ORGANIZATION_BLOCK "Blocco Organizzativo"
TITLE = "Main Program Sweep (Cycle)"
AUTHOR : MassimoZ
FAMILY : NovaSrl
VERSION : 0.1


VAR_TEMP
  OB1_EV_CLASS : BYTE ;	//Bits 0-3 = 1 (Coming event), Bits 4-7 = 1 (Event class 1)
  OB1_SCAN_1 : BYTE ;	//1 (Cold restart scan 1 of OB 1), 3 (Scan 2-n of OB 1)
  OB1_PRIORITY : BYTE ;	//1 (Priority of 1 is lowest)
  OB1_OB_NUMBR : BYTE ;	//1 (Organization block 1, OB1)
  OB1_RESERVED_1 : BYTE ;	//Reserved for system
  OB1_RESERVED_2 : BYTE ;	//Reserved for system
  OB1_PREV_CYCLE : INT ;	//Cycle time of previous OB1 scan (milliseconds)
  OB1_MIN_CYCLE : INT ;	//Minimum cycle time of OB1 (milliseconds)
  OB1_MAX_CYCLE : INT ;	//Maximum cycle time of OB1 (milliseconds)
  OB1_DATE_TIME : DATE_AND_TIME ;	//Date and time OB1 started
END_VAR
BEGIN
NETWORK
TITLE =Condizioni di Sicurezza OK
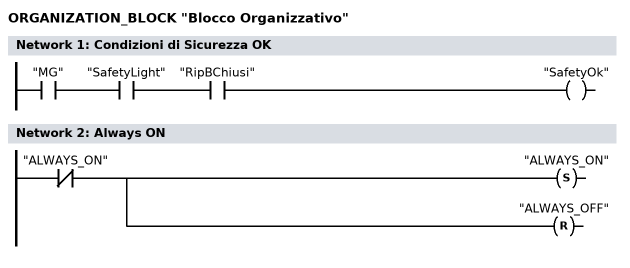
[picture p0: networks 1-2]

      U     "MG";
      U     "SafetyLight";
      U     "RipBChiusi";
      =     "SafetyOk";
NETWORK
TITLE =Always ON

      UN    "ALWAYS_ON";
      S     "ALWAYS_ON";
      R     "ALWAYS_OFF";
NETWORK
TITLE =Gestione Consensi

      UC    "Gest Consensi 2ndCC";

NETWORK
TITLE =Gestione Ciclo Automatico
//FC 49 gestisce il quadro di Ferrazza , mentre il FC50 gestisce, se abilitato,
//il quadro controllo corti tradizionale con slaughter STS
      UC    "Gest Auto 2ndCC";
// UC    "Gest Auto STS"
NETWORK
TITLE =Gestione Avvisi e Allarmi

      UC    "Gest Avvisi Allarmi";

NETWORK
TITLE =Gestione Interfaccia

      UC    "Gest Interfaccia";

NETWORK
TITLE =Gestione Output


      UC    "Gest Output 2ndCC";

NETWORK
TITLE =Gestione Trasmissione Dati Rete Supervisore alla Linea

      CALL "AG_SEND" (
           ACT                      := TRUE,
           ID                       := 1,
           LADDR                    := W#16#100,
           SEND                     := P#DB120.DBX10.0 BYTE 10,
           LEN                      := 10,
           DONE                     := "Gest Interfac Com Linea".Done,
           ERROR                    := "Gest Interfac Com Linea".ErrorTrasm,
           STATUS                   := "Gest Interfac Com Linea".StatusTrasm);

NETWORK
TITLE =Gestione Ricezione Dati Rete Supervisore da Linea

      CALL "AG_RECV" (
           ID                       := 1,
           LADDR                    := W#16#100,
           RECV                     := P#DB120.DBX0.0 BYTE 10,
           NDR                      := "Gest Interfac Com Linea".NDR,
           ERROR                    := "Gest Interfac Com Linea".ErrorRic,
           STATUS                   := "Gest Interfac Com Linea".StatusRic,
           LEN                      := "Gest Interfac Com Linea".LEN);

END_ORGANIZATION_BLOCK

